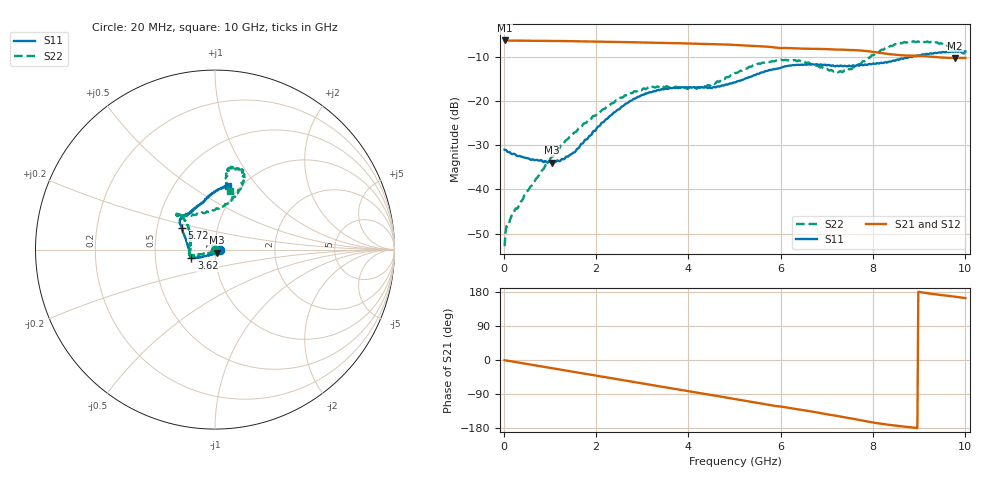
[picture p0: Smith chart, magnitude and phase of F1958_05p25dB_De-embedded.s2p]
! Integrated Device Technology
! Corporate Headquarters
! 6024 Silver Creek Valley Road
! San Jose, CA 95138  USA
! Phone:  1-408-284-8200
! Toll Free:  1-800-223-1366
! Webpage:  http://www.idt.com/
! Timing and RF Division
! 515 Groton Road, Suite 102
! Westford, MA 01886-6024
! Device:  F1958
! Description: 7-bit 0.25 dB Digital Step Attenuator
! Frequency:  0.001 -  6.000 GHz
! Package:  4x4 mm Thin QFN Plastic Package: 24 pin
! Ports:  2 RF, 12 DC
!  Pin  1  = D0
!  Pin  2  = VDD
!  Pin  3  = VMODE
!  Pin  4  = GND
!  Pin  5  = RF1  =  Port 1
!  Pin  6  = GND
!  Pin  7  = GND
!  Pin  8  = GND
!  Pin  9  = GND
!  Pin 10  = GND
!  Pin 11  = GND
!  Pin 12  = GND
!  Pin 13  = GND
!  Pin 14  = RF2  =  Port 2
!  Pin 15  = GND
!  Pin 16  = LE
!  Pin 17  = CLK
!  Pin 18  = DATA
!  Pin 19  = D6
!  Pin 20  = D5
!  Pin 21  = D4
!  Pin 22  = D3
!  Pin 23  = D2
!  Pin 24  = D1
! State:  21
! Atten State:  5.25 dB
! Voltage:  +3.30 Volts
! Current:  0.258 mA
! Data:  The device was measured on a F1958 evaluation board which has
!  individual transmission lines to the RF pins.  Data was collected
!  using a calibrated network analyzer.  The evaluation board was
!  de-embedded using Automatic Fixture Removal (AFR).
!  The reference plane is the edge of the package pin.
! Misc:
!  Action Tracker AT0419
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# GHz S dB R 50
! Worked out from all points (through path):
!   500 points, 20 MHz to 10 GHz, reference 50 ohm
!   highest |S21| = -6.31 dB at 20 MHz (marker M1); lowest = -10.3 dB at 9.78 GHz (marker M2)
!   group delay of S21, straight-line fit = 55.8 ps
!   lowest |S11| = -34.0 dB at 1.04 GHz (marker M3), VSWR 1.04, Z = 51 - j1.73 ohm
!   |S11| at or under -10 dB: start of sweep to 8.796 GHz; 8.803 GHz to 8.85 GHz (46.81 MHz wide, 0.53 % of centre)
!   |S22| runs from -52.9 to -6.5 dB; largest |S21 - S12| = 0.0012
!   S11 on the Smith chart (normalised r, x): 20 MHz: 1.06, -0.00; 3.62 GHz: 0.76, -0.07; 5.72 GHz: 0.67, +0.17; 10 GHz: 0.88, +0.72
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0.02  -31.02 -4.1  -6.31 -0.6  -6.31 -0.5  -52.86 -130.3
0.08  -31.47 -6.6  -6.33 -1.8  -6.33 -1.8  -48.36 -123.5
0.22  -31.95 -11.3  -6.35 -4.7  -6.35 -4.7  -45.36 -133.3
1.04  -33.98 -58.1  -6.41 -21.5  -6.41 -21.5  -32.62 -141.7
1.42  -32.34 -99.6  -6.46 -29.3  -6.46 -29.3  -28.19 -151.0
1.7  -29.64 -120.2  -6.50 -34.9  -6.50 -34.9  -25.62 -156.5
2.6  -21.05 -151.8  -6.67 -53.4  -6.66 -53.4  -19.01 -164.4
3.36  -17.54 -159.3  -6.86 -69.0  -6.86 -69.1  -16.86 -167.5
3.62  -17.09 -160.9  -6.90 -74.3  -6.91 -74.4  -16.69 -173.4
4.32  -16.98 -172.3  -7.06 -88.7  -7.07 -88.8  -16.67 161.2
5.02  -15.78 165.1  -7.31 -103.3  -7.32 -103.3  -13.65 138.3
5.72  -13.16 147.0  -7.73 -117.8  -7.74 -117.8  -11.13 135.5
6.28  -11.88 140.6  -8.08 -128.4  -8.10 -128.3  -10.77 137.4
6.68  -11.70 135.4  -8.19 -136.1  -8.21 -136.0  -11.64 133.0
7.1  -12.02 128.7  -8.32 -145.3  -8.33 -145.2  -13.01 116.0
7.38  -12.04 124.7  -8.41 -151.1  -8.42 -151.0  -13.08 95.0
7.9  -11.69 112.8  -8.75 -162.7  -8.75 -162.8  -10.26 71.7
8.34  -11.09 102.6  -9.38 -171.0  -9.38 -171.1  -7.83 67.2
8.76  -10.18 93.0  -9.73 -176.6  -9.73 -176.6  -6.58 70.5
9.24  -9.24 84.1  -9.96 175.0  -9.97 175.0  -6.71 78.3
9.78  -8.78 79.6  -10.29 167.0  -10.32 167.1  -8.10 80.2
10  -8.81 78.9  -10.25 163.3  -10.28 163.4  -9.49 75.9
